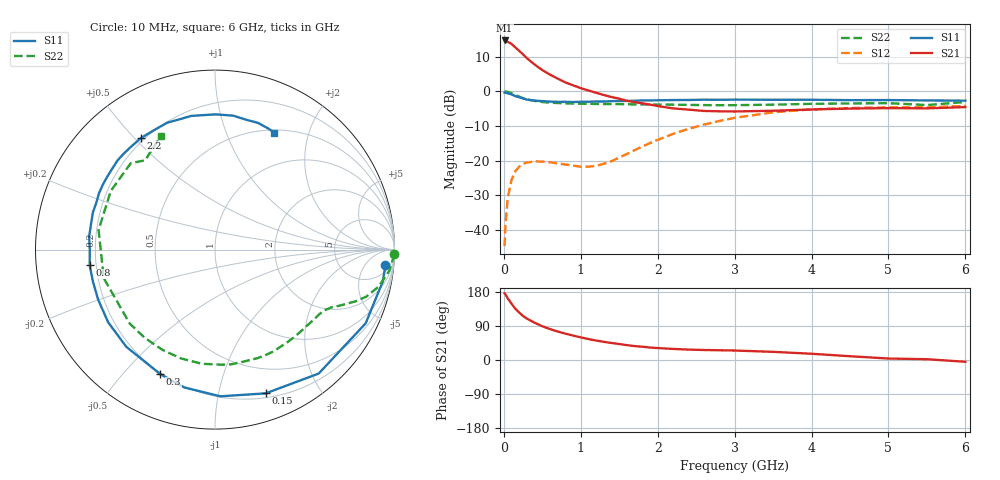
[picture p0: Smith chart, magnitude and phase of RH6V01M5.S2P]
! SIEMENS Small Signal Semiconductors
! BFR106
! Si NPN RF Bipolar Junction Transistor in SOT23
! VCE = 6 V  IC = 1.5 mA
! Common Emitter S-Parameters:  August  1996
# GHz  S  MA  R  50
!  f  S11  S21  S12  S22
! GHz  MAG  ANG  MAG  ANG  MAG  ANG  MAG  ANG
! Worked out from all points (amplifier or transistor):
!   36 points, 10 MHz to 6 GHz, reference 50 ohm
!   highest |S21| = 14.7 dB at 10 MHz (marker M1)
!   |S21| within 3 dB of that: start of sweep to 201 MHz
!   unconditionally stable (mu >= 1): 820.5 MHz to 1.813 GHz; 3.722 GHz to end of sweep
!   at 250 MHz: K = 0.29, MSG = 15.8 dB, |S12| = -21.0 dB
!   at 1.4 GHz: K = 1.30, MAG = 6.0 dB, |S12| = -20.2 dB
!   at 6 GHz: K = 1.02, MAG = -1.0 dB, |S12| = -4.3 dB
!   S11 on the Smith chart (normalised r, x): 10 MHz: 9, -17; 150 MHz: 0.24, -1.38; 300 MHz: 0.20, -0.63; 800 MHz: 0.17, -0.06; 2.2 GHz: 0.19, +0.52; 6 GHz: 0.53, +1.49
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0.01  0.9536 -5.2  5.407 176.0  0.0058 88.8  0.9989 -1.4
0.02  0.9518 -10.7  5.356 173.4  0.0114 84.9  0.9933 -2.9
0.05  0.9345 -26.1  5.184 162.8  0.0287 75.7  0.9784 -6.9
0.1  0.9004 -50.1  4.82 148.7  0.0525 63.5  0.934 -12.8
0.15  0.8492 -70.6  4.283 135.0  0.07 52.3  0.8824 -17.3
0.2  0.818 -87.9  3.837 125.2  0.0817 44.7  0.8366 -20.1
0.25  0.7869 -102.6  3.388 116.0  0.0893 38.2  0.7937 -22.3
0.3  0.7575 -113.8  2.99 109.2  0.0935 34.1  0.7653 -24.0
0.4  0.7332 -132.4  2.432 98.3  0.0971 27.7  0.7228 -26.5
0.5  0.7199 -145.8  2.019 89.0  0.0964 24.4  0.6978 -29.0
0.6  0.7083 -156.8  1.738 81.6  0.0944 23.0  0.6836 -31.8
0.8  0.7037 -172.9  1.341 69.5  0.0876 25.7  0.6684 -37.9
1.1  0.7053 168.2  1.024 55.2  0.0813 41.8  0.657 -48.5
1.6  0.7249 145.8  0.728 39.2  0.1244 71.5  0.6496 -68.6
2.2  0.7461 123.6  0.565 29.2  0.2422 73.3  0.6403 -96.6
2.8  0.7523 105.3  0.513 25.7  0.3718 60.8  0.6284 -128.7
3.5  0.7535 89.8  0.523 21.5  0.4965 42.9  0.6399 -165.6
4  0.7532 82.3  0.545 16.5  0.5476 30.4  0.6578 170.4
4.5  0.7439 76.3  0.562 9.9  0.5724 19.6  0.6662 150.6
5  0.7457 71.3  0.57 3.9  0.5846 10.8  0.6722 134.3
5.5  0.7369 66.2  0.566 2.1  0.5854 6.6  0.6318 128.0
6  0.7307 63.1  0.59 -4.7  0.6124 -1.6  0.6997 115.7
